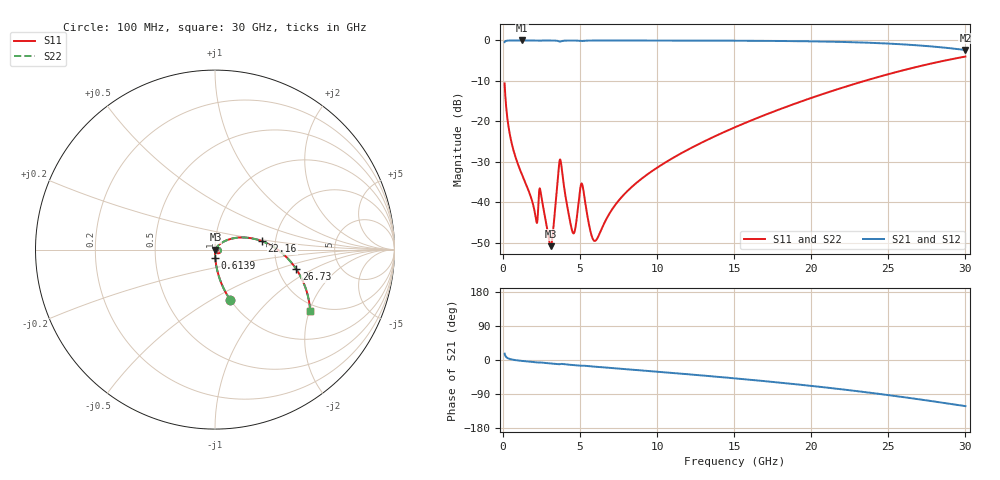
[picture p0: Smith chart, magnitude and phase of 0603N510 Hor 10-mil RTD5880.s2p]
# GHz S MA R 50
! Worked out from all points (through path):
!   3201 points, 100 MHz to 30 GHz, reference 50 ohm
!   highest |S21| = -0.01 dB at 1.24 GHz (marker M1); lowest = -2.4 dB at 30 GHz (marker M2)
!   group delay of S21, straight-line fit = 11 ps
!   lowest |S11| = -50.8 dB at 3.09 GHz (marker M3), VSWR 1.01, Z = 50.3 - j0.098 ohm
!   |S11| at or under -10 dB: start of sweep to 23.46 GHz
!   |S22| runs from -50.8 to -4.0 dB; largest |S21 - S12| = 0
!   S11 on the Smith chart (normalised r, x): 100 MHz: 1.00, -0.62; 613.9 MHz: 1.00, -0.10; 22.16 GHz: 1.70, +0.17; 26.73 GHz: 2.52, -0.70; 30 GHz: 1.78, -2.03
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0.1  0.2949 -73.1  0.9551 16.9  0.9551 16.9  0.2949 -73.1
0.361625  0.08427 -85.9  0.9959 3.8  0.9959 3.8  0.08427 -85.9
0.6139062  0.04881 -88.2  0.9981 1.0  0.9981 1.0  0.04881 -88.2
1.239937  0.02177 -89.6  0.9987 -2.4  0.9987 -2.4  0.02177 -89.6
2.11825  0.006497 -72.5  0.9974 -5.9  0.9974 -5.9  0.006497 -72.5
2.463969  0.01255 -69.0  0.9941 -6.7  0.9941 -6.7  0.01255 -69.0
3.09  0.002889 -19.7  0.9971 -9.1  0.9971 -9.1  0.002889 -19.7
3.230156  0.004152 22.2  0.9964 -9.7  0.9964 -9.7  0.004152 22.2
3.688  0.03373 -11.0  0.9662 -10.9  0.9662 -10.9  0.03373 -11.0
4.528937  0.004226 -33.1  0.996 -13.3  0.996 -13.3  0.004226 -33.1
4.697125  0.004917 1.9  0.9952 -14.0  0.9952 -14.0  0.004917 1.9
5.089563  0.01714 -17.5  0.9828 -15.0  0.9828 -15.0  0.01714 -17.5
5.687563  0.00427 -41.7  0.996 -16.7  0.996 -16.7  0.00427 -41.7
5.977219  0.003359 -4.9  0.9966 -17.7  0.9966 -17.7  0.003359 -4.9
7.612375  0.01119 51.5  0.9968 -23.0  0.9968 -23.0  0.01119 51.5
10.06978  0.02745 51.8  0.9961 -31.1  0.9961 -31.1  0.02745 51.8
15.05  0.08478 38.4  0.9915 -48.5  0.9915 -48.5  0.08478 38.4
20.03956  0.1962 19.6  0.9737 -68.5  0.9737 -68.5  0.1962 19.6
22.16059  0.2661 10.1  0.956 -78.2  0.956 -78.2  0.2661 10.1
25.01978  0.3839 -4.1  0.9136 -92.7  0.9136 -92.7  0.3839 -4.1
26.72969  0.4656 -13.5  0.8741 -102.2  0.8741 -102.2  0.4656 -13.5
30  0.6321 -32.9  0.7615 -121.7  0.7615 -121.7  0.6321 -32.9
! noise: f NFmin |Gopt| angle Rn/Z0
0.1  0.0002946  0.9191  0.3598  0.0008042
3.417  0.006906  0.8844  10.12  0.01286
6.743  0.00659  0.7761  19.89  0.005842
10.06  0.008628  0.7509  29.44  0.00654
13.39  0.01101  0.7445  38.81  0.007725
16.7  0.01368  0.7468  47.88  0.009112
20.03  0.01679  0.7555  56.69  0.01081
23.35  0.02055  0.7695  65.19  0.01298
26.67  0.02533  0.7882  73.45  0.01594
30  0.03169  0.811  81.47  0.02024
